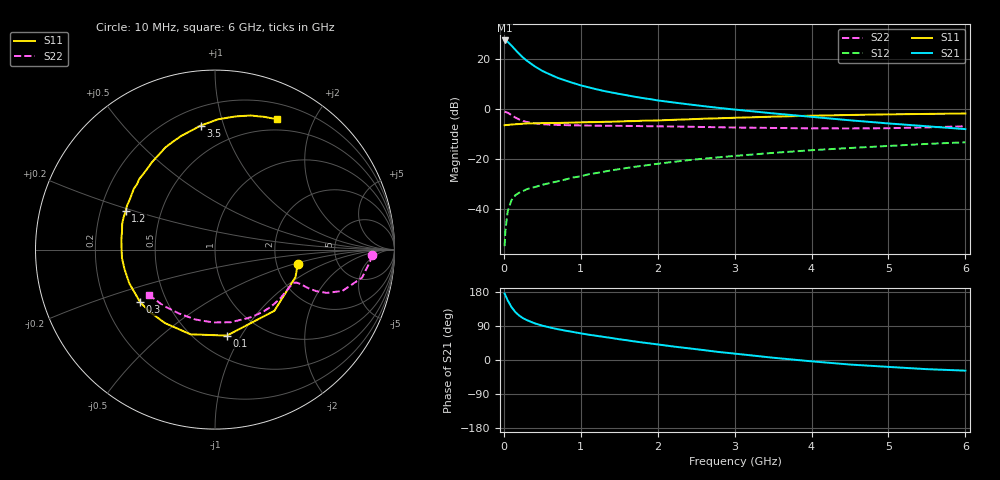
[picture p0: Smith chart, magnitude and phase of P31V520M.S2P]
! SIEMENS Small Signal Semiconductors
! BFP181
! Si NPN RF Bipolar Junction Transistor in SOT143
! VCE = 1.5 V  IC = 20 mA
! Common Emitter S-Parameters:  March  1996
# GHz  S  MA  R  50
!  f  S11  S21  S12  S22
! GHz  MAG  ANG  MAG  ANG  MAG  ANG  MAG  ANG
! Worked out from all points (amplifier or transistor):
!   36 points, 10 MHz to 6 GHz, reference 50 ohm
!   highest |S21| = 27.3 dB at 10 MHz (marker M1)
!   |S21| within 3 dB of that: start of sweep to 127.7 MHz
!   unconditionally stable (mu >= 1): start of sweep to 24.66 MHz; 263.2 MHz to end of sweep
!   at 250 MHz: K = 0.98, MSG = 26.7 dB, |S12| = -32.9 dB
!   at 1.4 GHz: K = 2.02, MAG = 9.8 dB, |S12| = -24.6 dB
!   at 6 GHz: K = 1.63, MAG = -2.0 dB, |S12| = -13.4 dB
!   S11 on the Smith chart (normalised r, x): 10 MHz: 2.63, -0.54; 100 MHz: 0.70, -0.87; 300 MHz: 0.35, -0.28; 1.2 GHz: 0.31, +0.19; 3.5 GHz: 0.31, +0.84; 6 GHz: 0.37, +1.52
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0.01  0.468 -9.9  23.14 175.3  0.0018 74.1  0.8744 -1.9
0.02  0.4739 -18.8  23.01 170.9  0.0036 80.6  0.8663 -4.4
0.05  0.4751 -45.9  21.76 157.4  0.009 75.2  0.8341 -10.8
0.1  0.4836 -82.1  18.24 139.4  0.015 58.2  0.7457 -18.0
0.15  0.4914 -106.1  15.03 126.4  0.0188 51.2  0.6676 -21.2
0.2  0.4953 -124.2  12.5 117.1  0.0211 48.7  0.6101 -22.3
0.25  0.5018 -135.8  10.53 110.2  0.0227 45.8  0.5693 -22.5
0.3  0.5096 -144.8  9.098 105.2  0.0248 46.0  0.5438 -22.3
0.4  0.5132 -158.5  7.063 96.8  0.0272 46.7  0.5114 -21.9
0.5  0.5159 -168.0  5.707 90.7  0.0303 47.6  0.4928 -22.0
0.6  0.5205 -174.9  4.846 85.8  0.0329 50.1  0.4819 -22.4
0.7  0.5206 179.1  4.147 81.4  0.0355 51.4  0.4754 -23.3
0.8  0.5247 173.8  3.669 77.5  0.0386 52.2  0.4712 -24.1
1.1  0.54 160.6  2.684 66.9  0.0491 54.8  0.4622 -28.0
1.2  0.542 156.5  2.461 64.0  0.0519 55.2  0.46 -29.7
1.7  0.5672 139.9  1.738 49.0  0.0693 55.3  0.4523 -38.1
2.2  0.6006 125.8  1.34 35.7  0.0868 53.1  0.4424 -47.8
2.8  0.6464 110.9  1.038 21.0  0.1075 49.3  0.4279 -60.8
3.5  0.6953 96.6  0.809 6.0  0.1315 44.3  0.4137 -77.9
4.5  0.7517 81.0  0.588 -12.0  0.1646 35.7  0.4046 -105.7
5.5  0.789 69.6  0.447 -24.2  0.1986 26.8  0.425 -132.8
6  0.8039 64.6  0.392 -28.1  0.2142 22.0  0.4463 -145.5
